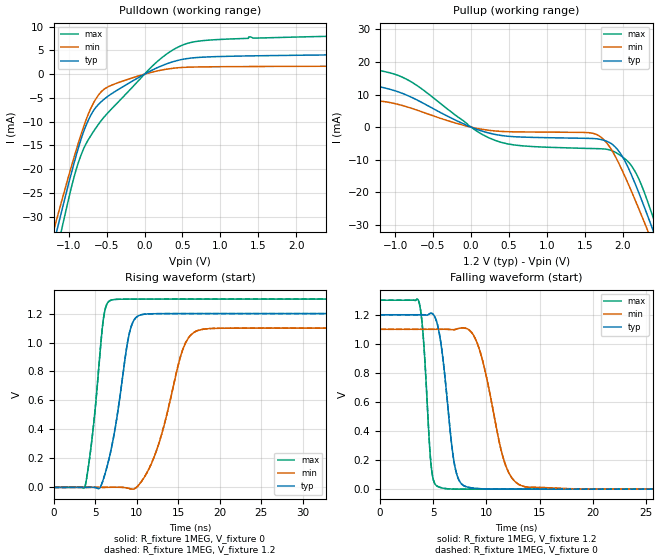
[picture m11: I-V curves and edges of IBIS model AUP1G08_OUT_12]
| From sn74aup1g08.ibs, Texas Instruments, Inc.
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[Model]   AUP1G08_OUT_12
Model_type  Output
Vref =   0
Rref =   1E6
Cref =   30p
Vmeas =   0.6
| variable   typ   min   max
C_comp   2.92pF   2.19pF   3.94pF
| C_pullup   3.08pF   2.19pF   3.94pF
| C_pulldown   2.75pF   2.30pF   3.24pF
[Temperature Range]   40   100   -40
| Ambient temperature   25   85   -40
[Voltage range]   1.2   1.1   1.3
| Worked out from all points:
|   slope of the pulldown table from 0 to 0.18 V, typ, clamps not added: 125 ohm
|   slope of the pullup table from 0 to 0.18 V, typ, clamps not added: 123 ohm
|   rising waveform, R_fixture 1MEG, V_fixture 0: 20-80 % time 1.94ns typ, 3ns min, 1.3ns max; typ from 0 V to 1.2 V
|   falling waveform, R_fixture 1MEG, V_fixture 1.2: 20-80 % time 1.04ns typ, 1.9ns min, 619ps max; typ from 1.2 V to 0 V
|   rising waveform, R_fixture 1MEG, V_fixture 1.2: 20-80 % time 1.94ns typ, 3ns min, 1.3ns max; typ from 0 V to 1.2 V
|   falling waveform, R_fixture 1MEG, V_fixture 0: 20-80 % time 1.04ns typ, 1.9ns min, 619ps max; typ from 1.2 V to 0 V
[Pulldown]
| AUP1G08_OUT_12
|   Voltage   I(typ)   I(min)   I(max)
-3.6V     -203.7mA   -186.7mA   -224.7mA
-1.215V   -36.79mA   -33.9mA    -41.57mA
-1.165V   -33.51mA   -30.94mA   -37.91mA
-1.12V    -30.59mA   -28.3mA    -34.64mA
-1.08V    -28.02mA   -25.97mA   -31.77mA
-930mV    -18.77mA   -17.54mA   -21.69mA
-835mV    -13.59mA   -12.6mA    -16.93mA
-695mV    -8.263mA   -6.752mA   -12.62mA
-560mV    -5.647mA   -3.536mA   -9.551mA
195mV     1.548mA    762.4uA    3.019mA
610mV     3.376mA    1.481mA    6.659mA
7.2V      4.761mA    1.852mA    9.574mA
[Pullup]
| AUP1G08_OUT_12
|   Voltage   I(typ)   I(min)   I(max)
-3.6V     26.64mA    8.231mA    37.82mA
-3.07V    21.45mA    10.47mA    31mA
-2.05V    13.05mA    7.514mA    19.68mA
-955mV    10.79mA    6.947mA    15.81mA
400mV     -2.561mA   -1.314mA   -4.679mA
1.61V     -3.491mA   -1.891mA   -6.566mA
1.87V     -5.388mA   -7.571mA   -7.321mA
2.095V    -13.5mA    -18.51mA   -11.17mA
2.33V     -27.18mA   -31.68mA   -22.8mA
2.44V     -34.09mA   -38.11mA   -30.26mA
2.505V    -38.25mA   -41.96mA   -34.83mA
7.2V      -371.3mA   -348.8mA   -398.8mA
[Ramp]
| AUP1G08_OUT_12
| variable   typ   min   max
dV/dt_r   0.72/1.96E-09   0.67/3.05E-09   0.78/1.31E-09
dV/dt_f   0.73/1.05E-09   0.67/1.92E-09   0.78/6.28E-10
R_load = 1MEG
[Rising Waveform]
| AUP1G08_OUT_12
R_fixture =   1MEG
C_fixture =   0
L_fixture =   0
V_fixture =   0
V_fixture_min = 0
V_fixture_max = 0
|   Time   V(typ)   V(min)   V(max)
0s        20.88nV    142.6nV    977.7pV
3.785ns   -65.38uV   -46.15nV   4.569mV
4.755ns   608.1uV    -587.2nV   396.4mV
5.995ns   55mV       -189.5uV   1.158V
6.815ns   229.9mV    610.9uV    1.29V
9.06ns    1.045V     -7.076mV   1.3V
10.3ns    1.187V     18.65mV    1.3V
15.59ns   1.2V       954.8mV    1.3V
17.07ns   1.2V       1.075V     1.3V
45ns      1.2V       1.1V       1.3V
[Falling Waveform]
| AUP1G08_OUT_12
R_fixture =   1MEG
C_fixture =   0
L_fixture =   0
V_fixture =   1.2
V_fixture_min = 1.1
V_fixture_max = 1.3
|   Time   V(typ)   V(min)   V(max)
0s        1.2V       1.1V       1.3V
3.65ns    1.2V       1.1V       1.291V
4.815ns   1.21V      1.1V       155.5mV
5.515ns   1.095V     1.1V       15.6mV
6.96ns    186.5mV    1.097V     678.2uV
8.02ns    18.93mV    1.108V     122.7uV
9.445ns   3.134mV    936.2mV    77.92uV
11.77ns   222.6uV    169.9mV    74.86uV
13.27ns   145.8uV    24.43mV    74.8uV
45ns      135uV      244.1uV    74.79uV
[Rising Waveform]
| AUP1G08_OUT_12
R_fixture =   1MEG
C_fixture =   0
L_fixture =   0
V_fixture =   1.2
V_fixture_min = 1.1
V_fixture_max = 1.3
|   Time   V(typ)   V(min)   V(max)
0s        135uV      244.2uV    74.83uV
3.785ns   69.67uV    244uV      4.703mV
4.755ns   741.6uV    243.5uV    397mV
5.995ns   55.43mV    54.69uV    1.158V
6.815ns   230.7mV    854.6uV    1.29V
9.055ns   1.045V     -6.735mV   1.3V
10.3ns    1.187V     19.34mV    1.3V
15.57ns   1.2V       954.7mV    1.3V
17.05ns   1.2V       1.075V     1.3V
45ns      1.2V       1.1V       1.3V
[Falling Waveform]
| AUP1G08_OUT_12
R_fixture =   1MEG
C_fixture =   0
L_fixture =   0
V_fixture =   0
V_fixture_min = 0
V_fixture_max = 0
|   Time   V(typ)   V(min)   V(max)
0s        1.2V       1.1V       1.3V
3.65ns    1.2V       1.1V       1.29V
4.815ns   1.21V      1.1V       155.2mV
5.51ns    1.096V     1.1V       15.66mV
6.96ns    186mV      1.097V     602.1uV
8.02ns    18.74mV    1.108V     47.72uV
9.445ns   2.972mV    935.3mV    3.071uV
11.77ns   87.28uV    170.1mV    31.97nV
13.27ns   10.62uV    24.12mV    -26.9nV
45ns      -23.96nV   116.7nV    -36.08nV
